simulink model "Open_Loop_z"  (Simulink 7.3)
settings: Solver=ode4  StartTime=0.0  StopTime=10  FixedStep=0.04  RelTol=1e-3
undefined symbols (not defined in the file or in its folder): Acz, Av4, Bcz, Bv4, Ccz, Cv4, Dcz, Dv4

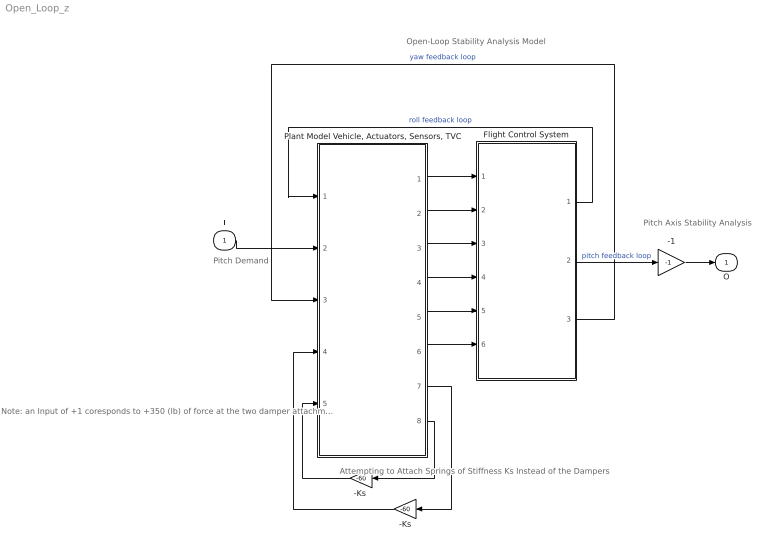
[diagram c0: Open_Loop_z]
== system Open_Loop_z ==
  note: Open-Loop Stability Analysis Model
  note: Pitch Axis Stability Analysis
  note: Pitch Demand
  note: Note: an Input of +1 coresponds to +350 (lb) of force at the two damper attachments because the vehicle model force inputs are normalized at 350 lb
  note: Attempting to Attach Springs of Stiffness Ks Instead of the Dampers
  I : Inport  OutDataType=sfix(16)  OutScaling=2^0
  -1 : Gain  Gain=-1  ParameterDataType=sfix(16)  ParameterScaling=2^0  OutDataType=sfix(16)  OutScaling=2^0
  -Ks : Gain  Gain=-60  ParameterDataType=sfix(16)  ParameterScaling=2^0  OutDataType=sfix(16)  OutScaling=2^0
  "-Ks " : Gain  Gain=-60  ParameterDataType=sfix(16)  ParameterScaling=2^0  OutDataType=sfix(16)  OutScaling=2^0
  Flight Control System : Subsystem
  "Plant Model Vehicle, Actuators, Sensors, TVC" : Subsystem
  O : Outport  OutDataType=sfix(16)  OutScaling=2^0
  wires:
  -1/1 -> O/1
  "Plant Model Vehicle, Actuators, Sensors, TVC"/1(phi) -> Flight Control System/1(Phi)
  "Plant Model Vehicle, Actuators, Sensors, TVC"/2(theta) -> Flight Control System/2(Theta)
  "Plant Model Vehicle, Actuators, Sensors, TVC"/3(psi) -> Flight Control System/3(Psi)
  "Plant Model Vehicle, Actuators, Sensors, TVC"/4(P) -> Flight Control System/4(P)
  "Plant Model Vehicle, Actuators, Sensors, TVC"/5(Q) -> Flight Control System/5(Q)
  "Plant Model Vehicle, Actuators, Sensors, TVC"/6(R) -> Flight Control System/6(R)
  -Ks/1 -> "Plant Model Vehicle, Actuators, Sensors, TVC"/4(F-left)
  "-Ks "/1 -> "Plant Model Vehicle, Actuators, Sensors, TVC"/5(F-right)
  "Plant Model Vehicle, Actuators, Sensors, TVC"/8(dZ-Rght) -> "-Ks "/1
  "Plant Model Vehicle, Actuators, Sensors, TVC"/7(dZ-Left) -> -Ks/1
  Flight Control System/1(DP-TVC) -> "Plant Model Vehicle, Actuators, Sensors, TVC"/1(DP)  "roll feedback loop"
  I/1 -> "Plant Model Vehicle, Actuators, Sensors, TVC"/2(DQ)
  Flight Control System/2(DQ-TVC) -> -1/1  "pitch feedback loop"
  Flight Control System/3(DR-TVC) -> "Plant Model Vehicle, Actuators, Sensors, TVC"/3(DR)  "yaw feedback loop"

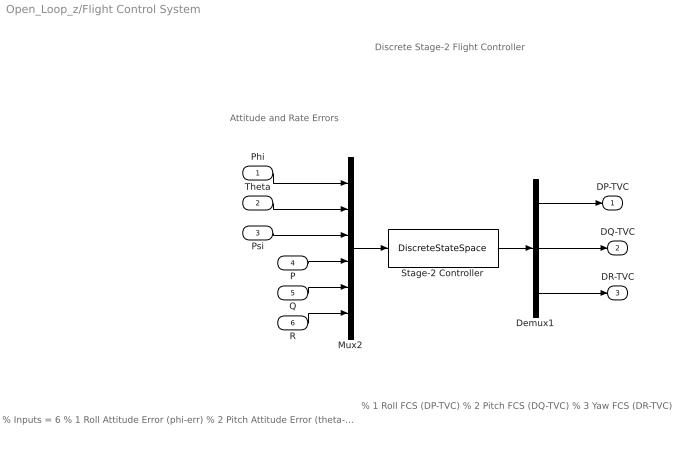
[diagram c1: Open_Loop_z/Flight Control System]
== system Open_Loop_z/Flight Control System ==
  note: Discrete Stage-2 Flight Controller
  note: Attitude and Rate Errors
  note: % Inputs = 6 % 1 Roll Attitude Error (phi-err) % 2 Pitch Attitude Error (theta-err) % 3 Yaw Attitude Error (psi-err) % 4 Roll Rate Error (p-err) % 5 Pitch Rate Error (q-err) % 6 Yaw Rate Error (r-err)
  note: % 1 Roll FCS (DP-TVC) % 2 Pitch FCS (DQ-TVC) % 3 Yaw FCS (DR-TVC)
  Phi : Inport  OutDataType=sfix(16)  OutScaling=2^0
  Theta : Inport  Port=2  OutDataType=sfix(16)  OutScaling=2^0
  Psi : Inport  Port=3  OutDataType=sfix(16)  OutScaling=2^0
  P : Inport  Port=4  OutDataType=sfix(16)  OutScaling=2^0
  Q : Inport  Port=5  OutDataType=sfix(16)  OutScaling=2^0
  R : Inport  Port=6  OutDataType=sfix(16)  OutScaling=2^0
  Demux1 : Demux  Outputs=3
  Mux2 : Mux  Inputs=6
  Stage-2 Controller : DiscreteStateSpace  A=Acz  B=Bcz  C=Ccz  D=Dcz  SampleTime=0.04
  DP-TVC : Outport  OutDataType=sfix(16)  OutScaling=2^0
  DQ-TVC : Outport  Port=2  OutDataType=sfix(16)  OutScaling=2^0
  DR-TVC : Outport  Port=3  OutDataType=sfix(16)  OutScaling=2^0
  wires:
  Q/1 -> Mux2/5
  R/1 -> Mux2/6
  Phi/1 -> Mux2/1
  Theta/1 -> Mux2/2
  Psi/1 -> Mux2/3
  Mux2/1 -> Stage-2 Controller/1
  Stage-2 Controller/1 -> Demux1/1
  P/1 -> Mux2/4
  Demux1/2 -> DQ-TVC/1
  Demux1/1 -> DP-TVC/1
  Demux1/3 -> DR-TVC/1

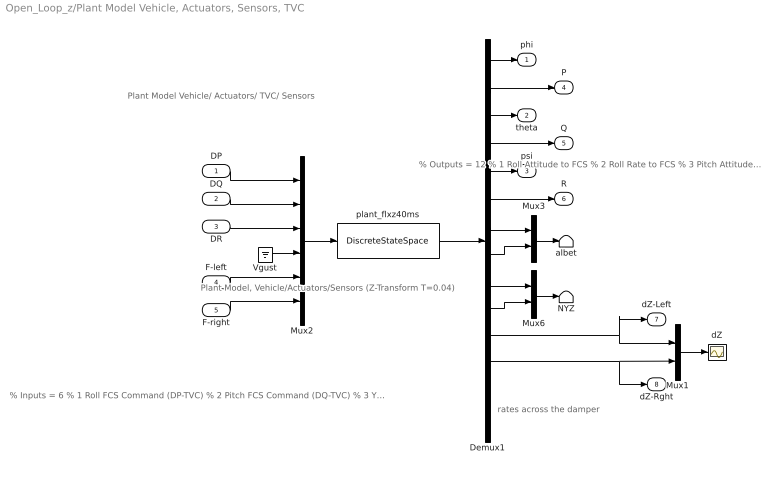
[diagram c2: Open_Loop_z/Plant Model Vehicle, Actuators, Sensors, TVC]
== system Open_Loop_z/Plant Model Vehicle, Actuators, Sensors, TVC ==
  note: Plant Model Vehicle/ Actuators/ TVC/ Sensors
  note: % Inputs = 6 % 1 Roll FCS Command (DP-TVC) % 2 Pitch FCS Command (DQ-TVC) % 3 Yaw FCS Command (DR-TVC) % 4 Wind-Gust Velocity (ft/sec) % 5 Left Coulomb Damper Force % 6 Right Coulomb Damper Force
  note: % Outputs = 12 % 1 Roll Attitude to FCS % 2 Roll Rate to FCS % 3 Pitch Attitude to FCS % 4 Pitch Rate to FCS % 5 Yaw Attitude to FCS % 6 Yaw Rate to FCS % 7 Angle of Attack, alpha (rad) % 8 Angle of Sideslip, beta (rad) % 9 Normal Accelerometer, Nz (ft/sec^2) % 10 Lateral Accelerometer, Ny (ft/sec^2) % 11 Left Damper Extension (ft) % 12 Right Damper Extension (ft) % 13 Left Damper Rate (ft/sec) % 14 Right Damper Rate (ft/s)
  note: rates across the damper
  note: Plant Model, Vehicle/Actuators/Sensors (Z-Transform T=0.04)
  DP : Inport  OutDataType=sfix(16)  OutScaling=2^0
  DQ : Inport  Port=2  OutDataType=sfix(16)  OutScaling=2^0
  DR : Inport  Port=3  OutDataType=sfix(16)  OutScaling=2^0
  F-left : Inport  Port=4  OutDataType=sfix(16)  OutScaling=2^0
  F-right : Inport  Port=5  OutDataType=sfix(16)  OutScaling=2^0
  Demux1 : Demux  Outputs=14
  Mux1 : Mux  Inputs=2
  Mux2 : Mux  Inputs=6
  Mux3 : Mux  Inputs=2
  Mux6 : Mux  Inputs=2
  NYZ : Terminator
  Vgust : Ground
  albet : Terminator
  dZ : Scope
  plant_flxz40ms : DiscreteStateSpace  A=Av4  B=Bv4  C=Cv4  D=Dv4  SampleTime=0.04
  phi : Outport  OutDataType=sfix(16)  OutScaling=2^0
  theta : Outport  Port=2  OutDataType=sfix(16)  OutScaling=2^0
  psi : Outport  Port=3  OutDataType=sfix(16)  OutScaling=2^0
  P : Outport  Port=4  OutDataType=sfix(16)  OutScaling=2^0
  Q : Outport  Port=5  OutDataType=sfix(16)  OutScaling=2^0
  R : Outport  Port=6  OutDataType=sfix(16)  OutScaling=2^0
  dZ-Left : Outport  Port=7  OutDataType=sfix(16)  OutScaling=2^0
  dZ-Rght : Outport  Port=8  OutDataType=sfix(16)  OutScaling=2^0
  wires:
  F-left/1 -> Mux2/5
  F-right/1 -> Mux2/6
  DP/1 -> Mux2/1
  DQ/1 -> Mux2/2
  DR/1 -> Mux2/3
  Demux1/7 -> Mux3/1
  Demux1/9 -> Mux6/1
  Mux2/1 -> plant_flxz40ms/1
  Mux3/1 -> albet/1
  Mux6/1 -> NYZ/1
  Vgust/1 -> Mux2/4
  Demux1/2 -> P/1
  Demux1/6 -> R/1
  Demux1/8 -> Mux3/2
  Demux1/10 -> Mux6/2
  plant_flxz40ms/1 -> Demux1/1
  Mux1/1 -> dZ/1
  Demux1/3 -> theta/1
  Demux1/1 -> phi/1
  Demux1/5 -> psi/1
  Demux1/4 -> Q/1
  Demux1/11 -> Mux1/1, dZ-Left/1
  Demux1/12 -> Mux1/2, dZ-Rght/1
